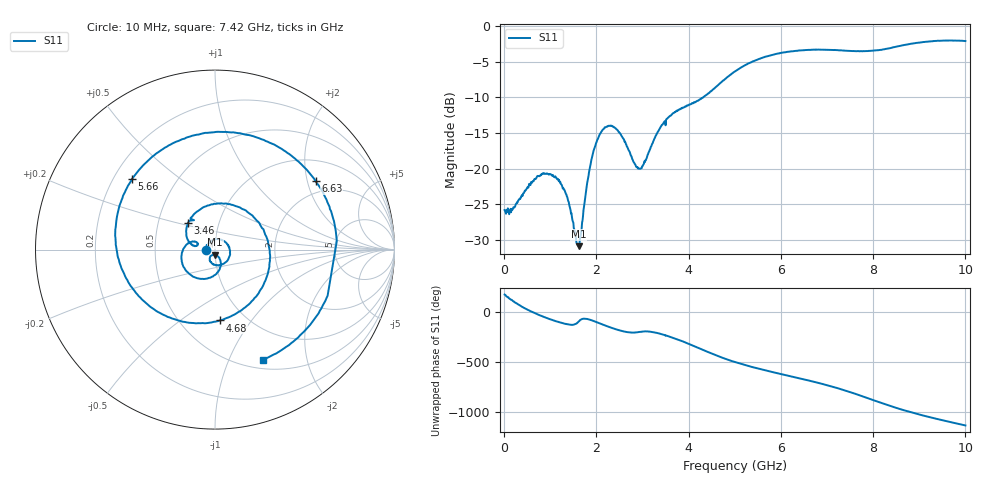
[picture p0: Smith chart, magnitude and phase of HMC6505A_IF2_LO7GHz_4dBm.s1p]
! Analog Devices, Inc.
! 1 Analog Way
! Wilmington, MA 01887
! http://www.analog.com
! Date:  2021-09-17 NN
! Board Name:  EV1HMC6505ALC5 (125487-1) with HMC6505ALC5 installed
! File Description:  S-Parameters for evaluation board without connectors or board loss de-embedded
! File Generation:  Calibrated Network Analyzer
! Chip Part Number:  HMC6505A
! Chip Description:  GaAs, MMIC, IQ Upconverter
! Chip Frequency:  5.5 to 8.6 GHz
! Chip Package:  LCC, 4.9 x 4.9 x 1 mm
! Chip State:
!  Temperature:  25C
!  LO Frequency:  7GHz
!  LO Power:  4dBm
! Note:
!  Analog Devices supplies this data as a sample of measured data at the evaluation board
!  ports for this product.  Your particular data for this product may vary.
!  Analog Devices reserves the right to change this data at anytime.
!  All lines below in this file are as is from the Network Analyzer.
!Keysight Technologies,N5245A,MY49151104,A.10.65.16
!Date: Tuesday, September 14, 2021 10:49:45
!Correction: S22(Full 2 Port(1,2))
!S1P File: Measurement: S22:
# Hz S  dB  R 50
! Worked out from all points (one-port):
!   980 points, 10 MHz to 10 GHz, reference 50 ohm
!   lowest |S11| = -30.9 dB at 1.62 GHz (marker M1), VSWR 1.06, Z = 50 - j2.86 ohm
!   |S11| at or under -10 dB: start of sweep to 4.316 GHz
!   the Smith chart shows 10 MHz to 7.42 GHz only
!   S11 on the Smith chart (normalised r, x): 10 MHz: 0.90, +0.00; 3.46 GHz: 0.71, +0.22; 4.68 GHz: 0.77, -0.72; 5.66 GHz: 0.28, +0.35; 6.63 GHz: 1.59, +2.25; 7.42 GHz: 0.60, -1.34
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1e7  -25.81 179.4
8.3e8  -20.73 -38.7
1.26e9  -22.51 -105.9
1.62e9  -30.86 -89.0
2e9  -16.34 -96.6
2.51e9  -15.03 179.2
2.94e9  -20.02 164.2
3.46e9  -13.56 135.8
3.76e9  -11.88 89.4
4.26e9  -10.22 -5.5
4.68e9  -8.06 -85.9
5.01e9  -6.35 -138.5
5.32e9  -5.21 179.6
5.66e9  -4.33 139.4
6.26e9  -3.56 74.5
6.63e9  -3.37 34.3
6.89e9  -3.34 4.1
7.1e9  -3.38 -22.3
7.14e9  -3.40 -27.6
7.42e9  -3.49 -66.7
7.51e9  -3.52 -80.2
7.79e9  -3.54 -124.6
8.13e9  -3.39 179.7
8.48e9  -2.96 125.8
8.76e9  -2.59 86.7
9.03e9  -2.33 52.7
9.38e9  -2.11 12.5
1e10  -2.14 -53.4
